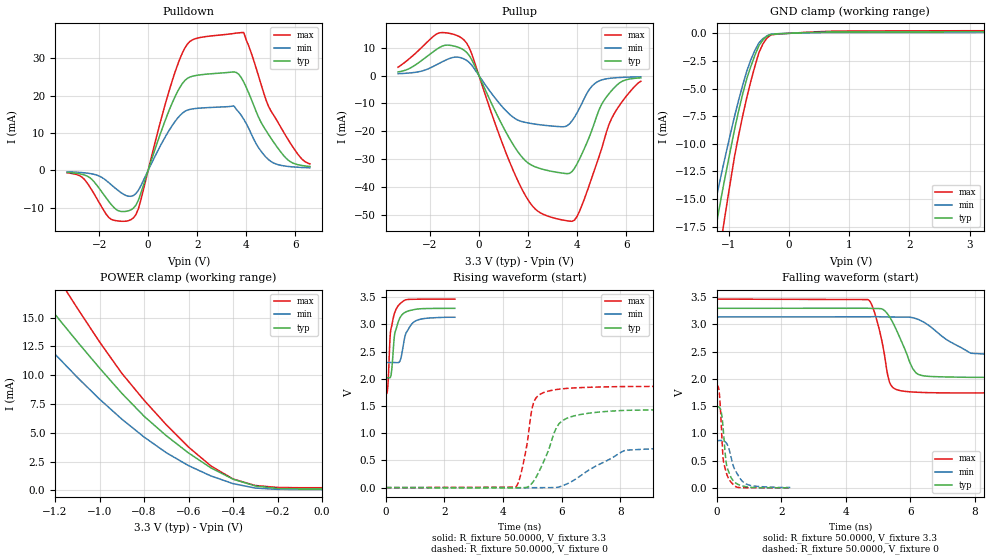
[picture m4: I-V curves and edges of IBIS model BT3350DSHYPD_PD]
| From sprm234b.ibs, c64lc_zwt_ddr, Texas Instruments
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[Model]   BT3350DSHYPD_PD
Model_type   I/O
Polarity   Non-Inverting
Enable   Active-Low
Vinl =  0.8V
Vinh =  2V
Cref =  15.0000pF
Rref =  100.0000M
Vref =  0V
Vmeas =  1.65
C_comp   1.471252p   1.436254p   1.510805p
[Model Spec]
Vinl   0.8V   0.8V   0.8V
Vinh   2V   2V   2V
[Temperature Range]   25   125   -40
[Voltage Range]   3.3   3.14   3.47
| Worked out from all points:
|   slope of the pulldown table from 0 to 0.495 V, typ, clamps not added: 50.8 ohm
|   slope of the pullup table from 0 to 0.495 V, typ, clamps not added: 51.2 ohm
|   GND clamp passes 1 mA (typ) near -0.48 V on its own axis
|   POWER clamp passes 1 mA (typ) near -0.40 V on its own axis
|   rising waveform, R_fixture 50.0000, V_fixture 3.3: 20-80 % time 200ps typ, 279ps min, 163ps max; typ from 2.02 V to 3.29 V
|   rising waveform, R_fixture 50.0000, V_fixture 0: 20-80 % time 703ps typ, 1.69ns min, 352ps max; typ from 0 V to 1.48 V
|   falling waveform, R_fixture 50.0000, V_fixture 3.3: 20-80 % time 553ps typ, 1.54ns min, 357ps max; typ from 3.3 V to 2.02 V
|   falling waveform, R_fixture 50.0000, V_fixture 0: 20-80 % time 185ps typ, 328ps min, 143ps max; typ from 1.49 V to 0.001 V
[POWER_clamp]
|   voltage   I(typ)   I(min)   I(max)
-3.3V     77.91mA    57.63mA    95.03mA
-1.433V   21.27mA    16.78mA    26.06mA
-1.267V   16.91mA    13.21mA    20.88mA
-1.133V   13.69mA    10.48mA    16.82mA
-900mV    8.425mA    6.184mA    10.16mA
-800mV    6.437mA    4.63mA     7.826mA
-600mV    3.248mA    2.149mA    3.759mA
-500mV    1.961mA    1.259mA    2.13mA
-400mV    975.9uA    588.8uA    987.5uA
-300mV    386.7uA    204.1uA    427.4uA
-200mV    168.8uA    89.69uA    256.3uA
0V        135.2uA    73.11uA    232.2uA
[Pulldown]
|   voltage   I(typ)   I(min)   I(max)
-3.3V     -544.2uA   -373.8uA   -649.3uA
-2.6V     -1.226mA   -645.1uA   -2.397mA
-1.5V     -9.17mA    -3.874mA   -13.14mA
-600mV    -10.12mA   -6.727mA   -12.73mA
-300mV    -6.174mA   -4.15mA    -8.052mA
900mV     16.8mA     11.19mA    22.28mA
1.5V      24.11mA    15.83mA    32.83mA
3.5V      26.39mA    17.27mA    36.71mA
3.8V      24.86mA    14.73mA    36.94mA
5V        8.733mA    2.435mA    16.05mA
5.8V      2.332mA    999.4uA    7.304mA
6.6V      1.052mA    693.5uA    1.743mA
[Pullup]
|   voltage   I(typ)   I(min)   I(max)
-3.3V     1.324mA    694.3uA    3.024mA
-1.7V     9.62mA     4.052mA    15.11mA
-600mV    9.081mA    5.972mA    12.73mA
1.1V      -20.32mA   -12.63mA   -27.71mA
1.9V      -30.67mA   -16.84mA   -43.22mA
2.5V      -33.44mA   -17.7mA    -49.34mA
3.7V      -35.15mA   -17.28mA   -52.38mA
4.1V      -30.02mA   -11.73mA   -48.83mA
4.6V      -19.78mA   -3.879mA   -36.81mA
5.2V      -7.671mA   -1.145mA   -20.29mA
5.7V      -2.836mA   -700.2uA   -11.11mA
6.6V      -790.1uA   -430.1uA   -2.018mA
[GND_clamp]
|   voltage   I(typ)   I(min)   I(max)
-3.3V     -92.33mA   -69.21mA   -111.6mA
-1.3V     -20.32mA   -17.24mA   -25.07mA
-1.233V   -18.17mA   -15.53mA   -22.64mA
-1.167V   -16.1mA    -13.84mA   -20.23mA
-1.1V     -14.11mA   -12.16mA   -17.83mA
-1.033V   -12.23mA   -10.54mA   -15.49mA
-900mV    -8.592mA   -7.411mA   -11mA
-700mV    -4.086mA   -3.393mA   -5.792mA
-500mV    -1.121mA   -867.3uA   -1.756mA
-366.7mV  -263.7uA   -227.4uA   -427.7uA
633.3mV   110.1uA    61.95uA    173.6uA
3.233V    135uA      75.49uA    231.1uA
[Ramp]
| variable   typ   min   max
dV/dt_f  0.7714886/0.5567375n  0.5147355/1.320253n   1.05043/0.3592928n
dV/dt_r  0.8952337/0.7082026n  0.5210426/1.67516n   1.134422/0.3511887n
R_load = 50
[Rising Waveform]
R_fixture = 50.0000
V_fixture = 3.3
V_fixture_min = 3.14
V_fixture_max = 3.47
|   time   V(typ)   V(min)   V(max)
0s        2.017V     2.297V     1.725V
60ps      2.019V     2.3V       1.822V
135ps     2.019V     2.3V       2.695V
165ps     2.045V     2.3V       2.897V
300ps     2.824V     2.299V     3.215V
420ps     3.045V     2.299V     3.343V
510ps     3.148V     2.373V     3.392V
675ps     3.227V     2.825V     3.451V
945ps     3.27V      3.04V      3.462V
2.355ns   3.295V     3.131V     3.465V
[Rising Waveform]
R_fixture = 50.0000
V_fixture = 0
V_fixture_min = 0
V_fixture_max = 0
|   time   V(typ)   V(min)   V(max)
0s        52.09uV    29.54uV    82.66uV
4.425ns   -3.312mV   -74.72uV   9.189mV
4.635ns   -131.6uV   -2.364mV   305.3mV
4.995ns   84.05mV    -1.094mV   1.461V
5.13ns    193.1mV    -523.1uV   1.65V
5.925ns   1.182V     14.59mV    1.81V
7.05ns    1.376V     361mV      1.846V
8.175ns   1.42V      687.4mV    1.858V
17.14ns   1.47V      842.1mV    1.872V
115.9ns   1.482V     860.7mV    1.883V
[Falling Waveform]
R_fixture = 50.0000
V_fixture = 3.3
V_fixture_min = 3.14
V_fixture_max = 3.47
|   time   V(typ)   V(min)   V(max)
0s        3.297V     3.138V     3.465V
4.695ns   3.297V     3.141V     3.455V
4.98ns    3.293V     3.142V     3.043V
5.31ns    3.182V     3.137V     2.047V
5.415ns   3.085V     3.137V     1.874V
6.075ns   2.191V     3.125V     1.76V
6.555ns   2.048V     2.991V     1.749V
7.875ns   2.03V      2.472V     1.743V
12.63ns   2.026V     2.304V     1.75V
122ns     2.024V     2.293V     1.726V
[Falling Waveform]
R_fixture = 50.0000
V_fixture = 0
V_fixture_min = 0
V_fixture_max = 0
|   time   V(typ)   V(min)   V(max)
0s        1.489V     868mV      1.884V
60ps      1.487V     868.5mV    1.826V
90ps      1.473V     869.5mV    1.672V
150ps     1.358V     870.3mV    1.047V
210ps     1.014V     863.8mV    481mV
300ps     433.5mV    822.8mV    271.5mV
420ps     219.4mV    623.6mV    122.6mV
555ps     104.6mV    342mV      38.41mV
900ps     22.34mV    74.49mV    3.04mV
2.28ns    1.466mV    6.49mV     347.4uV
